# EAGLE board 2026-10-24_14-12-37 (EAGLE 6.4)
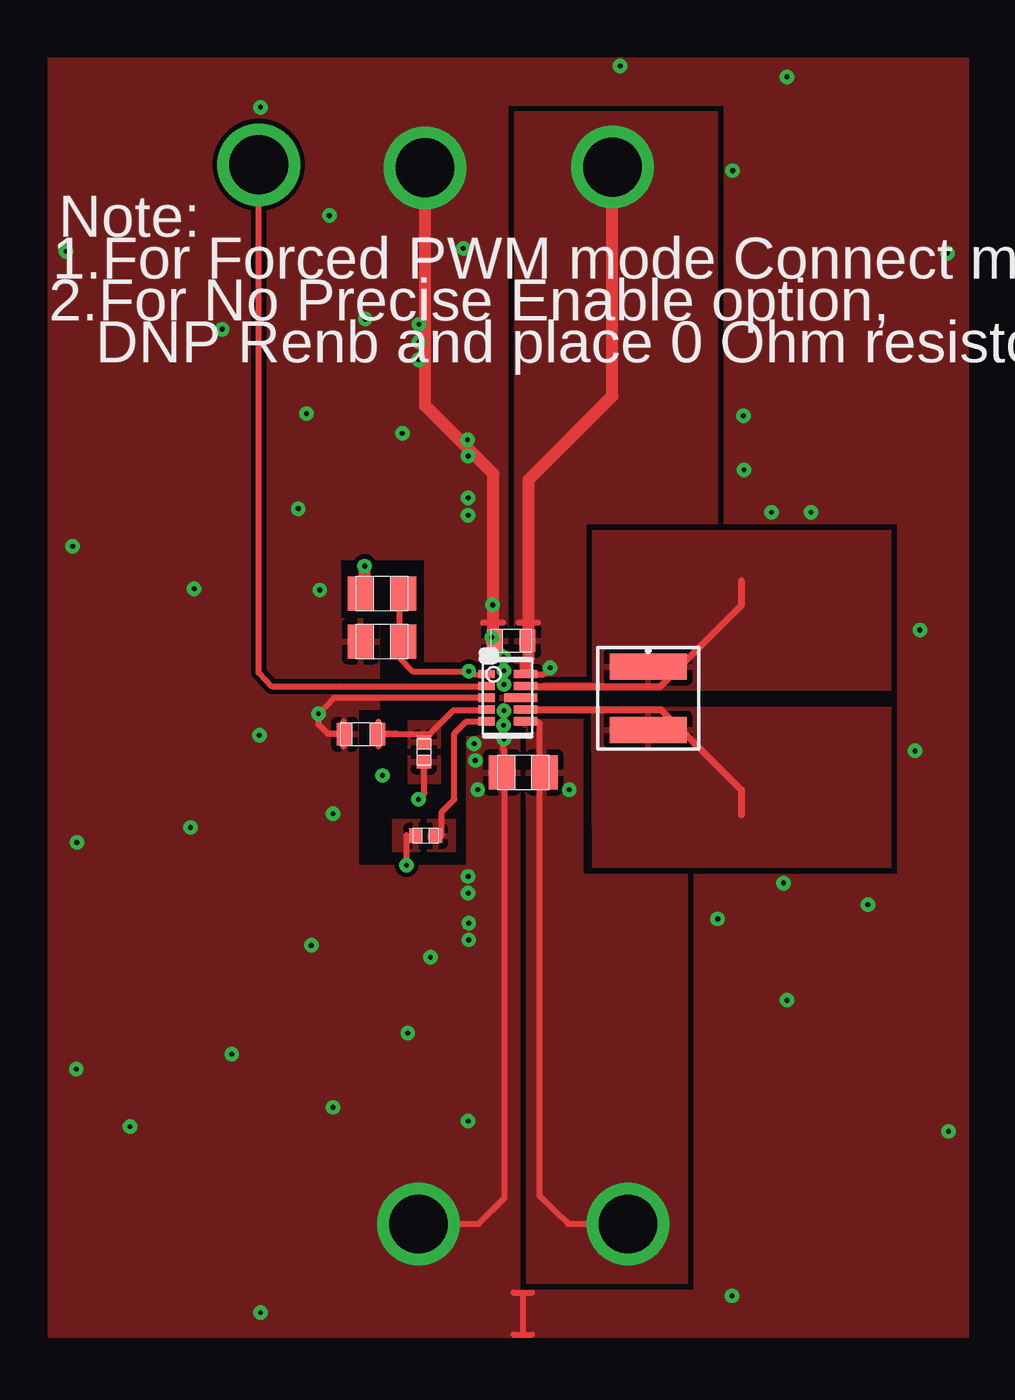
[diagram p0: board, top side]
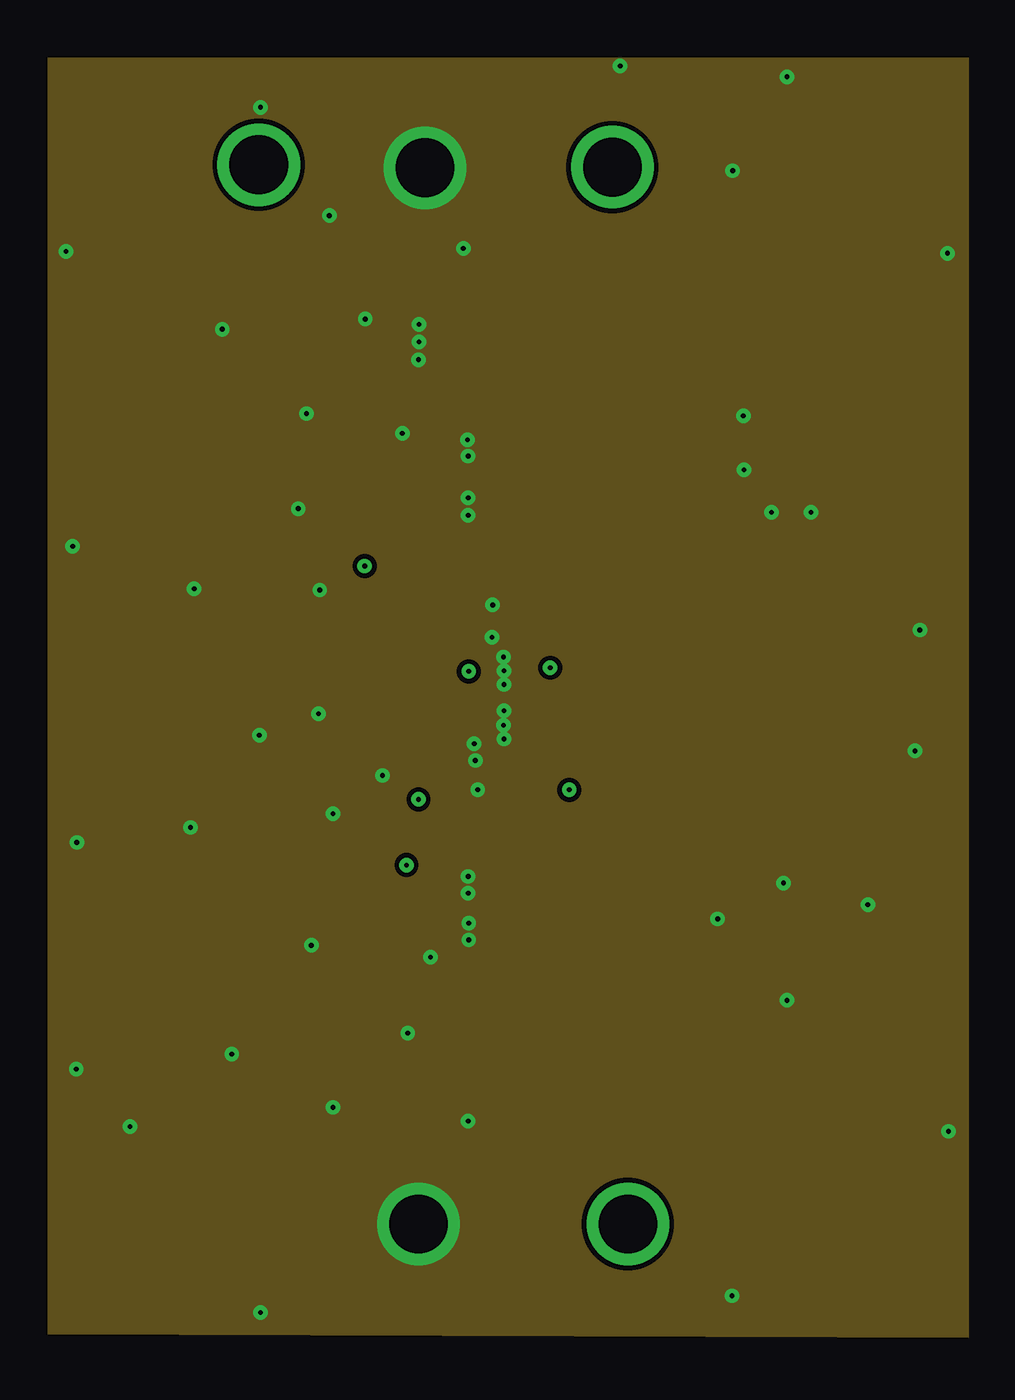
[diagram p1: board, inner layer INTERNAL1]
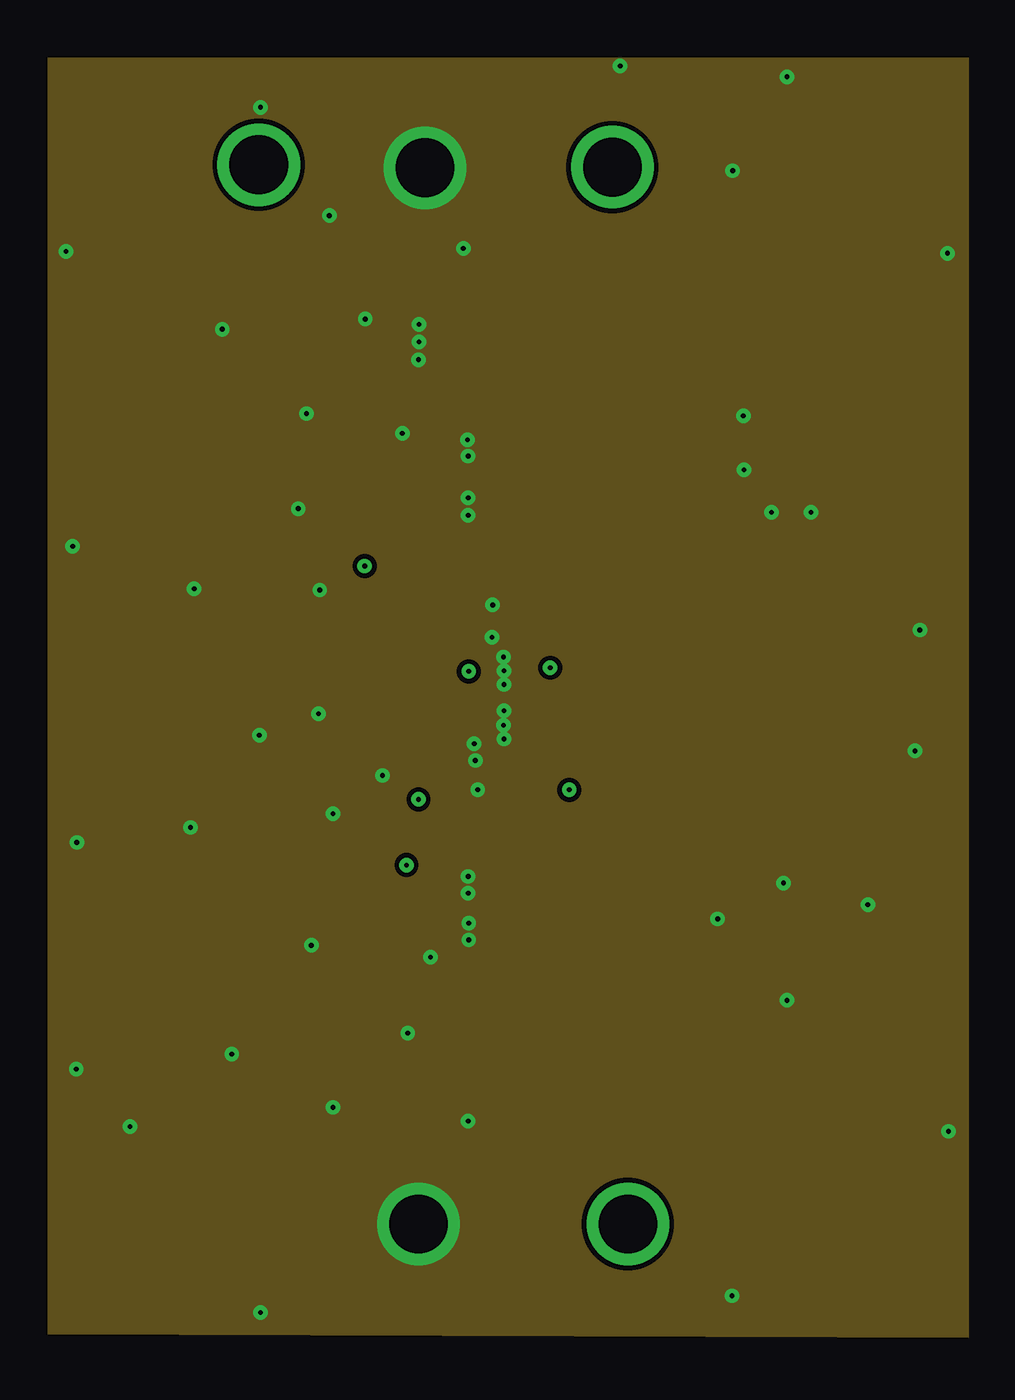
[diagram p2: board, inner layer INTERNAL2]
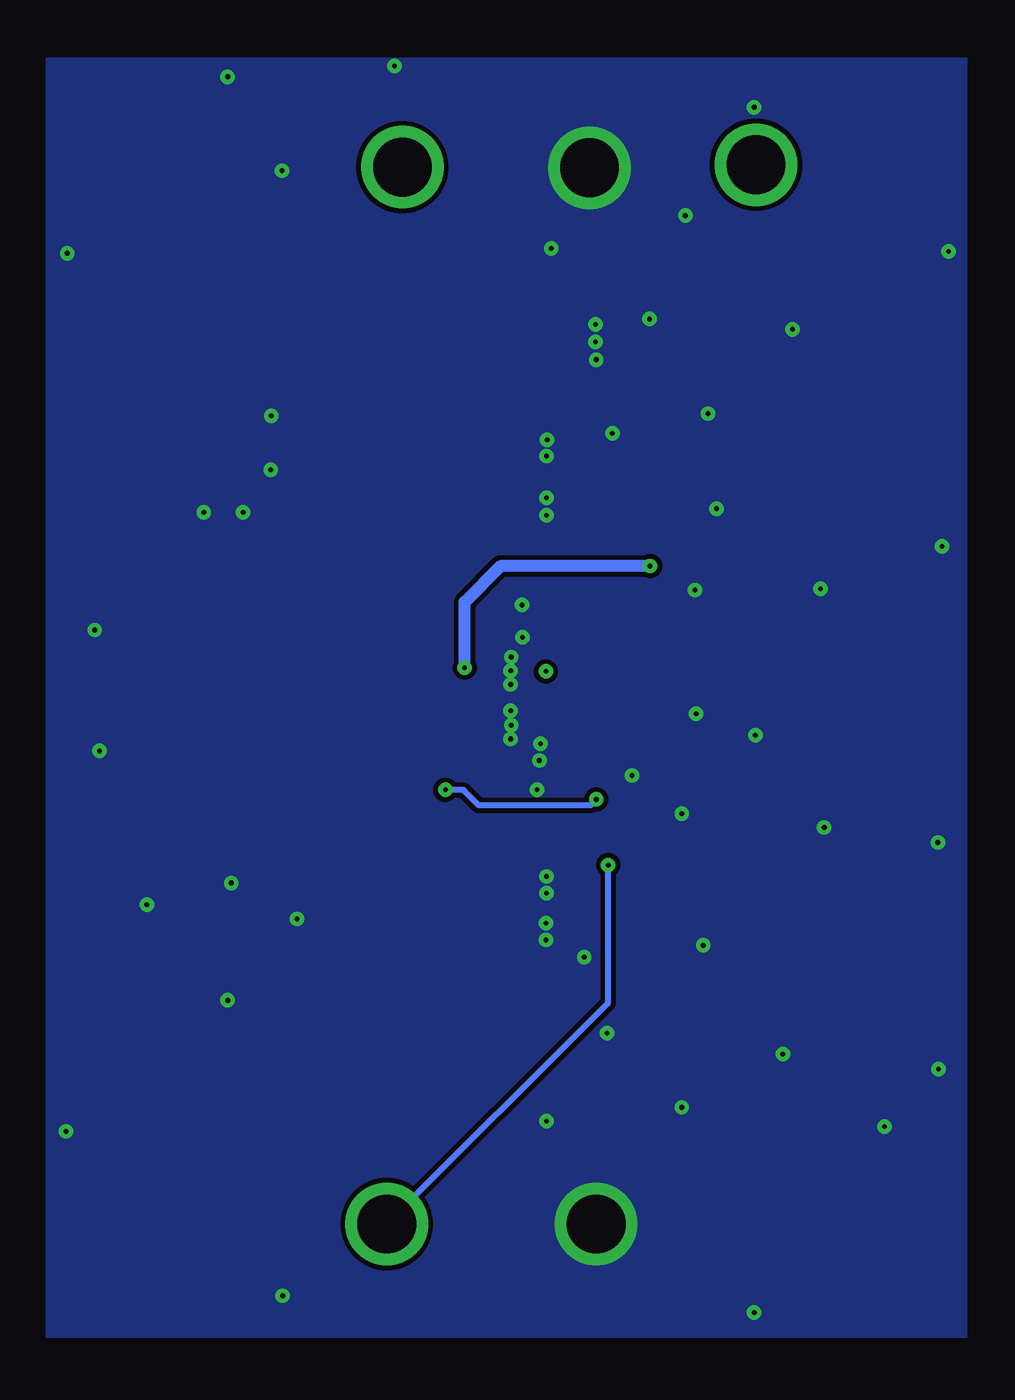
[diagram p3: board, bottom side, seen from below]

No outline drawn. Coordinates in mm, seen from the top.
Copper layers ((1*2)+(15*16)): TOP / INTERNAL1 / layer 15 / BOTTOM

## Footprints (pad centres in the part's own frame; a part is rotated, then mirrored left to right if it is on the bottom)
0603 = smd 0.66 x 0.965: 1 -0.699,0; 2 0.699,0
0805 = smd 1.118 x 1.448: 1 -0.902,0; 2 0.902,0
TP-1502 = drill 0.813 pad 1.651 round: 1 0,0
XFL4015 = smd 1.118 x 3.251: 1 -1.346,0; 2 1.346,0
0402 = smd 0.559 x 0.61: 1 -0.419,0; 2 0.419,0
DLA0010A = smd 0.7 x 0.35: 1 -0.9,1; 2 -0.9,0.5; 3 -0.9,0; 4 -0.9,-0.5; 5 -0.9,-1 | smd 1 x 0.35: 6 0.75,-1; 7 0.75,-0.5; 9 0.75,0.5; 10 0.75,1 | smd 1.4 x 0.35: 8 0.55,0

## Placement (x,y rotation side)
Cin  [0603]  45.85,55.75 180 top
Cout  [0805]  46.35,50.16 180 top
GND  [TP-1502]  42.19,75.82 270 top
GND1  [TP-1502]  41.88,30.99 270 top
L1  [XFL4015]  51.66,53.31 270 top
MODE  [TP-1502]  35.1,75.95 270 top
Renb  [0805]  40.36,55.73 180 top
Rent  [0805]  40.36,57.76 0 top
Rfbb  [0603]  39.47,51.79 180 top
Rfbt  [0402]  42.14,51.03 90 top
Rpg  [0402]  42.21,47.47 0 top
U1  [DLA0010A]  45.69,53.34 0 top
VIN  [TP-1502]  50.14,75.84 270 top
VOUT  [TP-1502]  50.8,30.99 270 top

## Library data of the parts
Cin = ultra-librarian; RefDes: Cin; Type: GRM188R60J226MEA0D
Cout = ultra-librarian; RefDes: Cout; Type: MSASL219LB5226MTNA01
GND = ultra-librarian; RefDes: GND; Type: TP-1502
GND1 = ultra-librarian; RefDes: GND1; Type: TP-1502
L1 = ultra-librarian; RefDes: L1; Type: XFL4015-471MEB
MODE = ultra-librarian; RefDes: MODE; Type: TP-1502
Renb = ultra-librarian; RefDes: Renb; Type: ERJ-6ENF1003V
Rent = ultra-librarian; RefDes: Rent; Type: ERJ-6ENF1003V
Rfbb = ultra-librarian; RefDes: Rfbb; Type: RC0603FR-0791KL
Rfbt = ultra-librarian; RefDes: Rfbt; Type: CRCW0402511KFKED
Rpg = ultra-librarian; RefDes: Rpg; Type: CRCW0402100KFKED
U1 = ultra-librarian; RefDes: U1; Type: TPS63802DLAR
VIN = ultra-librarian; RefDes: VIN; Type: TP-1502
VOUT = ultra-librarian; RefDes: VOUT; Type: TP-1502

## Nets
0: Cin.2 Cout.2 GND1.1 GND.1 Renb.2 Rfbb.2 U1.3 U1.8
2: Cin.1 Renb.1 Rent.1 Rent.2 U1.1 U1.10 VIN.1
5: Rfbb.1 Rfbt.2 U1.4
7: Cout.1 Rfbt.1 Rpg.1 U1.6 VOUT.1
9: L1.2 U1.7
10: Rpg.2 U1.5
11: MODE.1 U1.2
13: L1.1 U1.9

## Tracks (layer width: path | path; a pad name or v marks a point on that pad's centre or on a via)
0  (via drill 0.2 pad 0.48, 0.2 pad 0.61, 2.49 pad 3.48)
  TOP 0.254: 44.81,53.34 38.33,53.34 v37.67,52.65 37.67,52.2 38.05,51.82 38.73,51.82 | 45.95,26.29 46.35,26.29 | 46.35,26.29 46.74,26.29 | 46.35,28.07 46.74,28.07 | 45.95,28.07 46.35,28.07 | 46.35,26.29 46.35,28.07 | v41.91,30.99 44.45,30.99 45.57,32.11 45.57,49.51 45.57,51.08 45.52,51.13 45.52,51.61 | 45.44,51.92 45.57,51.92 | 45.44,51.71 45.44,52.17 | 45.57,51.71 45.57,52.17 | 38.72,51.28 38.72,52.32 | 44.65,56.53 45.49,56.53 | 44.63,53.33 44.96,53.33 | 45.74,53.33 46.79,53.33
  TOP 0.508: 42.19,65.73 45.09,62.84 45.09,56.54 45.09,55.52 v45.52,55.07 45.54,55.07 | 42.19,65.73 v42.19,75.84 | 42.19,65.73 42.55,65.41 | 45.52,51.61 v45.54,51.59 | 45.54,52.17
  other vias: 45.54,53.9 45.54,52.78 44.02,61.82 41.94,69.19 45.54,54.48 56.9,61.21 57.4,45.47 62.99,51.08 44.32,50.67 29.67,35.13 27.38,37.57 35.2,27.23 33.99,38.2 38.28,35.94 27.41,47.19 32.23,47.83 37.36,42.82 35.15,51.74 38.28,48.41 41.45,39.09 44.02,35.36 42.42,42.32 40.39,50.04 44.02,45.75 44.04,43.05 44.02,45.03 44.04,43.76 32.38,57.96 27.23,59.77 36.8,61.37 33.58,68.99 26.95,72.29 35.2,78.41 37.16,65.41 38.13,73.81 39.65,69.42 37.72,57.91 43.99,64.29 44.02,61.09 44.02,63.6 41.22,64.57 41.91,67.69 41.94,68.45 43.81,72.42 44.42,49.43 44.27,51.38 45.52,52.17 55.22,27.94 54.61,43.94 64.41,34.92 57.56,40.49 60.99,44.55 45.03,55.91 45.06,57.28 58.57,61.21 63.2,56.21 55.73,63.02 50.47,80.16 55.24,75.72 55.7,65.3 57.56,79.71 64.36,72.21
  pour TOP: 45.34,51.82 45.72,51.69 46.23,51.69 46.23,26.16 26.16,26.16 26.16,80.52 65.28,80.52 65.28,26.16 46.48,26.16 46.48,28.19 53.59,28.19 53.59,45.85 62.23,45.85 62.23,60.71 54.86,60.71 54.86,78.49 45.72,78.49 45.72,53.47 46.86,53.21 45.72,53.21 45.72,52.07 45.34,52.07 45.34,54.86 42.16,54.86 42.16,59.18 38.61,59.18 38.61,56.69 40.26,56.69 40.26,52.83 39.37,52.83 39.37,46.23 43.94,46.23 43.94,51.69
  pour BOTTOM (rank 6): 65.28,80.52 26.16,80.52 26.16,26.16 65.28,26.16
  pour INTERNAL2 (rank 5): 65.28,80.52 65.28,26.16 26.16,26.31 26.16,80.52
  pour INTERNAL1 (rank 6): 26.16,26.31 26.16,80.52 65.28,80.52 65.28,26.16
2  (via drill 0.2 pad 0.48, 2.49 pad 3.48)
  TOP 0.203: v44.04,54.46 44.17,54.33 44.81,54.33
  TOP 0.254: v39.62,58.93 39.62,58.9 | 41.12,57.78 | 41.12,57.78 41.12,55.75 41.15,55.73 41.15,54.99 41.66,54.46 v44.04,54.46 | v47.5,54.61 47.22,54.33 46.46,54.33 | 46.15,56.53 46.99,56.53 | 44.63,54.32 44.96,54.32 | 46.13,54.32 46.76,54.32
  TOP 0.508: 39.62,57.78 39.62,58.9 | 46.46,54.43 46.46,54.86 46.58,54.99 46.58,56.54 46.58,62.59 50.14,66.14 v50.14,75.87
  BOTTOM 0.508: v47.5,54.61 47.5,57.4 45.97,58.93 v39.62,58.93
  pour TOP (rank 5): 45.97,54.23 45.97,78.23 54.61,78.23 54.61,60.71 49.02,60.71 49.02,55.4 49.02,54.23
5
  TOP 0.254: 41,51.79 41,51.82 40.23,51.82 40.26,51.79 41,51.79 | 41,51.79 42.16,51.79 42.39,51.79 43.41,52.81 44.81,52.81 | 40.22,51.28 40.22,52.32 | 44.63,52.82 44.96,52.82
  pour TOP: 41.45,51.18 41.45,52.37 42.85,52.37 42.85,51.18
7  (via drill 0.2 pad 0.61, 2.49 pad 3.48)
  TOP 0.254: VOUT.1 48.26,30.99 47.07,32.16 47.07,49.51 47.07,52.22 46.97,52.32 46.46,52.32 | v41.91,49.02 42.16,49.28 42.16,50.29 | v41.4,46.23 41.4,47.5 | v41.4,46.23 | 46.13,52.31 46.76,52.31
  BOTTOM 0.254: v41.91,49.02 42.14,48.77 46.89,48.77 47.55,49.43 v48.31,49.43 | VOUT.1 41.4,40.39 v41.4,46.23
  other vias: 50.8,30.99
  pour TOP: 41.45,49.68 41.45,50.88 42.85,50.88 42.85,49.68
  pour TOP (rank 2): 46.46,48.79 46.46,50.19 47.65,50.19 47.65,48.79
  pour TOP (rank 3): 40.79,46.79 40.79,48.18 41.99,48.18 41.99,46.79
  pour TOP (rank 4): 53.34,45.85 48.9,45.85 48.9,52.45 46.1,52.45 46.1,52.07 46.48,52.07 46.48,28.45 48.46,28.45 53.34,28.45
9
  TOP 0.254: 46.13,52.82 46.76,52.82
  TOP 0.305: 55.63,48.36 55.63,49.4 52.2,52.83 46.46,52.83
  pour TOP (rank 4): 61.98,46.1 49.28,46.1 49.25,52.7 46.02,52.93 47.93,52.93 61.98,52.93
10
  TOP 0.254: 42.9,47.5 42.9,48.49 43.43,49.02 43.43,51.82 43.94,52.32 44.81,52.32 | 44.63,52.31 44.96,52.31
  pour TOP (rank 2): 42.29,46.79 42.29,48.18 43.48,48.18 43.48,46.79
11  (via drill 2.49 pad 3.48)
  TOP 0.254: v35.13,75.97 35.13,57.33 35.13,54.41 35.69,53.82 38.61,53.82 44.81,53.82 | 44.63,53.81 44.96,53.81
13
  TOP 0.254: 46.13,53.81 46.76,53.81
  TOP 0.305: 46.46,53.82 52.17,53.82 55.63,57.28 55.63,58.29
  pour TOP (rank 3): 47.37,54 49.28,54 49.28,60.45 61.98,60.45 61.98,53.64 46.81,53.64 46.81,54

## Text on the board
ASSYNOTES: Note: | 1.For Forced PWM mode Connect mode TP to Vin TP. | 2.For No Precise Enable option, | DNP Renb and place 0 Ohm resistor for Rent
